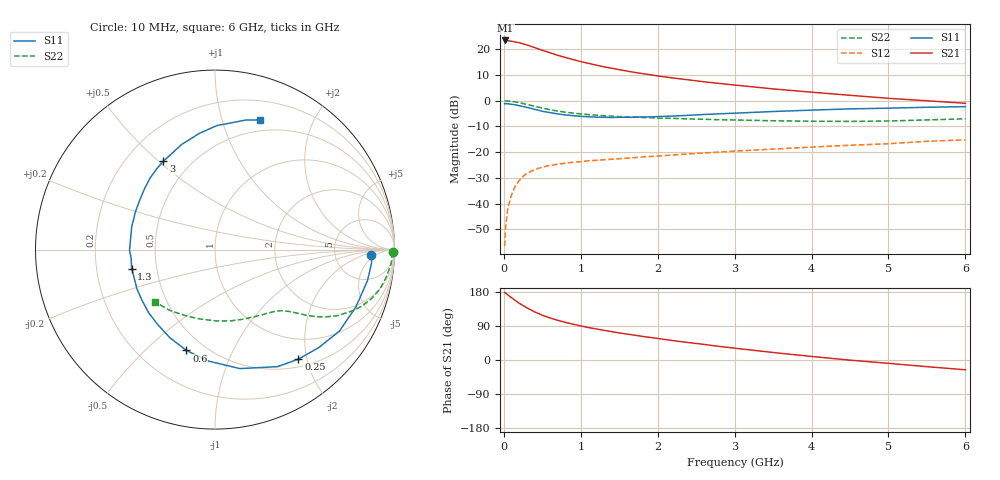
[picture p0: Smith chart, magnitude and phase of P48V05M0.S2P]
! SIEMENS Small Signal Semiconductors
! BFP182
! Si NPN RF Bipolar Junction Transistor in SOT143
! VCE = 8 V  IC = 5 mA
! Common Emitter S-Parameters:  March  1996
# GHz  S  MA  R  50
!  f  S11  S21  S12  S22
! GHz  MAG  ANG  MAG  ANG  MAG  ANG  MAG  ANG
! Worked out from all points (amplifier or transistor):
!   36 points, 10 MHz to 6 GHz, reference 50 ohm
!   highest |S21| = 23.3 dB at 20 MHz (marker M1)
!   |S21| within 3 dB of that: start of sweep to 422.2 MHz
!   unconditionally stable (mu >= 1): 1.666 GHz to 5.737 GHz
!   at 250 MHz: K = 0.21, MSG = 25.7 dB, |S12| = -29.4 dB
!   at 1.4 GHz: K = 0.91, MSG = 17.7 dB, |S12| = -22.8 dB
!   at 6 GHz: K = 0.97, MSG = 7.1 dB, |S12| = -15.2 dB
!   lowest NFmin = 1.25 dB at 450 MHz
!   S11 on the Smith chart (normalised r, x): 10 MHz: 14, -4; 250 MHz: 0.62, -1.85; 600 MHz: 0.40, -0.68; 1.3 GHz: 0.36, -0.10; 3 GHz: 0.35, +0.52; 6 GHz: 0.38, +1.33
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0.01  0.8713 -2.1  14.65 178.2  0.0015 86.3  0.9896 -0.9
0.02  0.8756 -4.8  14.69 177.0  0.0031 86.0  0.9876 -1.9
0.05  0.8673 -11.4  14.53 172.0  0.0079 85.4  0.9845 -4.7
0.1  0.8475 -22.1  14.19 164.4  0.0149 77.3  0.9656 -9.3
0.15  0.829 -33.1  13.72 157.0  0.0223 72.0  0.9439 -13.6
0.2  0.7959 -43.1  13.28 149.8  0.0282 67.4  0.9137 -17.4
0.25  0.7671 -52.7  12.65 143.3  0.0338 62.8  0.8786 -20.9
0.3  0.7393 -61.9  12.03 137.8  0.0387 59.2  0.8422 -23.8
0.4  0.6773 -78.2  10.68 127.0  0.0459 52.4  0.7762 -28.3
0.5  0.6219 -93.5  9.461 118.2  0.0513 46.9  0.7169 -31.6
0.6  0.584 -105.8  8.501 111.0  0.0555 43.4  0.6664 -34.0
0.7  0.5522 -116.9  7.555 104.8  0.0582 40.6  0.6273 -35.7
0.8  0.5264 -127.0  6.873 99.3  0.0612 38.8  0.5959 -37.0
1.1  0.4865 -153.5  5.293 85.6  0.0681 35.2  0.5355 -40.0
1.3  0.4766 -167.1  4.535 78.4  0.0712 33.9  0.5088 -42.0
1.7  0.476 169.3  3.528 65.5  0.0785 33.0  0.4771 -46.4
2.2  0.5012 147.1  2.743 51.2  0.0882 32.2  0.4521 -53.1
3  0.5701 120.4  2.004 31.2  0.1047 30.0  0.4204 -67.0
3.5  0.6145 107.6  1.687 19.8  0.1145 27.7  0.4067 -77.2
4.5  0.6912 89.1  1.268 -0.4  0.136 23.1  0.395 -101.1
5.5  0.7428 76.5  0.993 -17.6  0.1623 18.2  0.4221 -126.5
6  0.7646 70.9  0.888 -25.8  0.1735 14.2  0.4432 -138.9
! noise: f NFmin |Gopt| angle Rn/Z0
0.45  1.25  0.25  39  0.3
0.9  1.4  0.25  78  0.23
1.8  1.95  0.21  151  0.2
